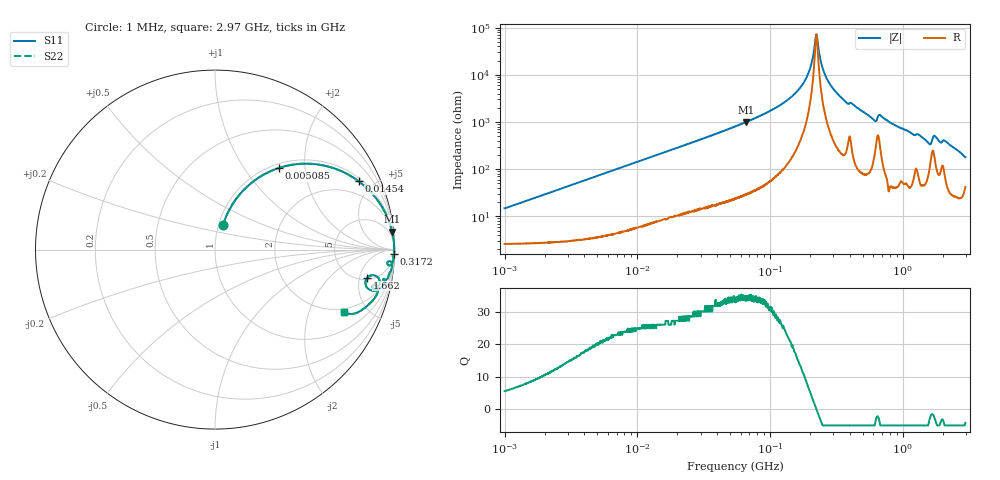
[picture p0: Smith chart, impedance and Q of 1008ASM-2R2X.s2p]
!s-Parameter Generated by FASTRON Sdn. Bhd.
!FASTRON P/N : 1008ASM-2R2X
!Keysight Technologies: E4991B_MY54100416_A.01.15
!Date: Tue Nov 21 10:08:19 2023
!Version  :Rev00  Wed Nov 22 15:09:02 2023
!Data & Calibration Information:
!Freq  S11  S21  S12  S22
!PortZ  Port1:50+j0  Port2:50+j0
!When reading reference impedance value at option line is always used.
! Remarks : This data is being provided solely for informational purposes.
# Hz S dB R 50
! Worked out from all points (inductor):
!   1599 points, 1 MHz to 2.97 GHz, reference 50 ohm
!   read as one part in series: L = 2.31 uH near 1.036 MHz
!   highest Q = 34.9 at 65.58 MHz (marker M1), where L = 2.41 uH
!   self-resonance near 223.5 MHz
!   S11 on the Smith chart (normalised r, x): 1 MHz: 1.05, +0.29; 5.085 MHz: 1.07, +1.46; 14.54 MHz: 1.16, +4.13; 317.2 MHz: 7, -83; 1.662 GHz: 5.42, -6.61; 2.97 GHz: 1.83, -3.50
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1000000  -16.90 71.8  -0.31 -8.1  -0.31 -8.1  -16.90 71.8
3804036  -6.56 58.7  -1.35 -28.0  -1.35 -28.0  -6.56 58.7
5084992  -4.77 51.9  -2.07 -35.2  -2.07 -35.2  -4.77 51.9
1.439846e7  -1.06 25.6  -7.29 -62.2  -7.29 -62.2  -1.06 25.6
1.454328e7  -1.04 25.4  -7.36 -62.4  -7.36 -62.4  -1.04 25.4
5.477226e7  -0.10 7.1  -18.20 -81.2  -18.20 -81.2  -0.10 7.1
6.558369e7  -0.07 5.8  -20.00 -82.6  -20.00 -82.6  -0.07 5.8
1.475212e8  -0.02 1.6  -31.00 -85.5  -31.00 -85.5  -0.02 1.6
1.829372e8  -0.01 0.8  -37.50 -83.4  -37.50 -83.4  -0.01 0.8
2.073156e8  -0.01 0.3  -45.60 -74.2  -45.60 -74.2  -0.01 0.3
2.19047e8  -0.01 0.1  -54.30 -45.3  -54.30 -45.3  -0.01 0.1
2.257233e8  -0.01 -0.0  -56.60 21.0  -56.60 21.0  -0.01 -0.0
2.558035e8  -0.01 -0.5  -41.00 80.1  -41.00 80.1  -0.01 -0.5
3.172153e8  -0.02 -1.4  -32.40 84.6  -32.40 84.6  -0.02 -1.4
6.079533e8  -0.15 -5.1  -21.00 76.2  -21.00 76.2  -0.15 -5.1
6.753166e8  -0.15 -3.9  -23.10 73.7  -23.10 73.7  -0.15 -3.9
7.846996e8  -0.07 -5.6  -20.20 82.5  -20.20 82.5  -0.07 -5.6
1.565327e9  -0.80 -14.6  -11.80 63.0  -11.80 63.0  -0.80 -14.6
1.662201e9  -1.28 -10.4  -13.20 45.9  -13.20 45.9  -1.28 -10.4
1.747494e9  -0.66 -10.0  -14.70 61.5  -14.70 61.5  -0.66 -10.0
2.199798e9  -0.57 -15.4  -11.50 68.6  -11.50 68.6  -0.57 -15.4
2.970126e9  -1.95 -25.6  -7.06 51.0  -7.06 51.0  -1.95 -25.6
